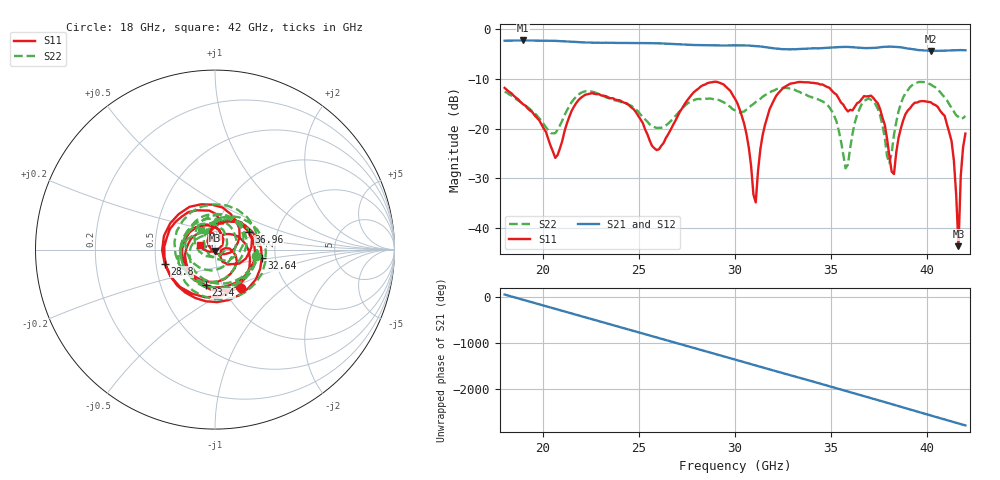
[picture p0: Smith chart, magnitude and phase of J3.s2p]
!Agilent Technologies,N5230A,US43500212,A.07.50.67
!Agilent N5230A: A.07.50.67
!Date: Monday, September 22, 2025 05:45:18
!Correction: S11(Full 2 Port(1,2))
!S21(Full 2 Port(1,2))
!S12(Full 2 Port(1,2))
!S22(Full 2 Port(1,2))
!S2P File: Measurements: S11, S21, S12, S22:
# Hz S  dB  R 50
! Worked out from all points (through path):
!   201 points, 18 GHz to 42 GHz, reference 50 ohm
!   highest |S21| = -2.33 dB at 18.96 GHz (marker M1); lowest = -4.4 dB at 40.2 GHz (marker M2)
!   lowest |S11| = -43.6 dB at 41.64 GHz (marker M3), VSWR 1.01, Z = 50 - j0.661 ohm
!   |S11| at or under -10 dB: start of sweep to end of sweep
!   |S22| runs from -28.0 to -10.6 dB; largest |S21 - S12| = 0.0064
!   S11 on the Smith chart (normalised r, x): 18 GHz: 1.20, -0.54; 23.4 GHz: 0.84, -0.35; 28.8 GHz: 0.56, -0.10; 32.64 GHz: 1.69, -0.18; 36.96 GHz: 1.43, +0.29; 42 GHz: 0.84, +0.04
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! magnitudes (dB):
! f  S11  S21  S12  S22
! 18 GHz  -11.8  -2.4  -2.4  -12.6
! 18.96 GHz  -15.1  -2.3  -2.3  -15.1
! 20.64 GHz  -25.9  -2.4  -2.4  -20.9
! 22.08 GHz  -13.6  -2.7  -2.7  -12.7
! 23.4 GHz  -13.8  -2.8  -2.8  -13.9
! 26.04 GHz  -24.2  -2.9  -2.9  -19.9
! 28.8 GHz  -10.7  -3.3  -3.3  -14.0
! 30 GHz  -14.0  -3.3  -3.3  -16.3
! 31.08 GHz  -34.8  -3.5  -3.5  -14.7
! 31.56 GHz  -19.3  -3.7  -3.7  -13.3
! 32.64 GHz  -11.5  -4.1  -4.1  -11.8
! 34.08 GHz  -10.8  -3.9  -3.9  -13.9
! 35.76 GHz  -16.0  -3.6  -3.6  -28.0
! 36.96 GHz  -13.5  -3.9  -3.9  -13.9
! 38.04 GHz  -25.5  -3.6  -3.6  -27.0
! 38.28 GHz  -29.1  -3.6  -3.6  -21.3
! 38.76 GHz  -18.4  -3.8  -3.8  -13.8
! 40.2 GHz  -14.7  -4.4  -4.4  -11.2
! 41.28 GHz  -22.5  -4.3  -4.3  -15.9
! 41.64 GHz  -43.6  -4.3  -4.3  -17.7
! 41.76 GHz  -29.4  -4.3  -4.3  -18.1
! 42 GHz  -21.0  -4.3  -4.3  -17.5
